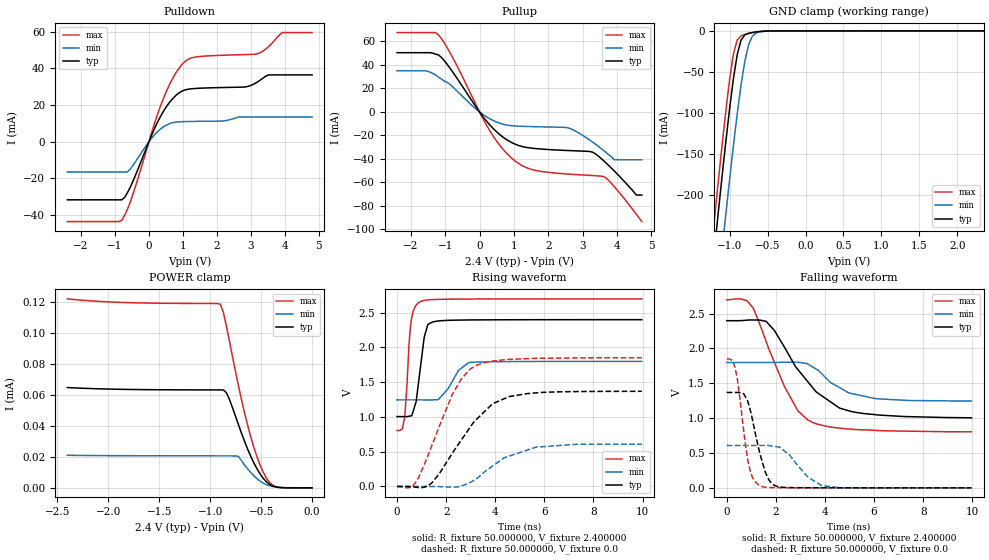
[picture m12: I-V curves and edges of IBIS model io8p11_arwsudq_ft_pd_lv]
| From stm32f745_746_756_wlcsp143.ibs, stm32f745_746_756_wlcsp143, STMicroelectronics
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|   Model io8p11_arwsudq_ft_pd_lv
[Model]  io8p11_arwsudq_ft_pd_lv
Model_type I/O
Polarity   Non-Inverting
Enable   Active-Low
Vinl =   0.720000V
Vinh =   1.680000V
Vmeas =  1.200000V
Cref =   30.000000pF
Rref =   100.000000M
Vref =   0.0V
C_comp   2.828100pF   2.774600pF   2.917100pF
[Temperature Range]   25.000000   0.125000k   -40.000000
[Pullup Reference]   2.400000V   1.800000V   2.700000V
[Pulldown Reference]   0.0V   0.0V   0.0V
[POWER Clamp Reference]   2.400000V   1.800000V   2.700000V
[GND Clamp Reference]   0.0V   0.0V   0.0V
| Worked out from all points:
|   slope of the pulldown table from 0 to 0.36 V, typ, clamps not added: 25 ohm
|   slope of the pullup table from 0 to 0.36 V, typ, clamps not added: 27.7 ohm
|   GND clamp passes 1 mA (typ) near -0.62 V on its own axis
|   rising waveform, R_fixture 50.000000, V_fixture 2.400000: 20-80 % time 296ps typ, 618ps min, 206ps max; typ from 1 V to 2.4 V
|   rising waveform, R_fixture 50.000000, V_fixture 0.0: 20-80 % time 1.73ns typ, 1.71ns min, 1.33ns max; typ from 0 V to 1.37 V
|   falling waveform, R_fixture 50.000000, V_fixture 2.400000: 20-80 % time 1.84ns typ, 1.34ns min, 1.4ns max; typ from 2.4 V to 1 V
|   falling waveform, R_fixture 50.000000, V_fixture 0.0: 20-80 % time 556ps typ, 948ps min, 410ps max; typ from 1.37 V to 0 V
[Pulldown]
|Voltage   I(typ)   I(min)   I(max)
-2.4V     -31.67mA   -16.51mA   -43.52mA
-800mV    -31.67mA   -16.51mA   -42.86mA
-480mV    -21.98mA   -13.17mA   -29.21mA
80mV      3.63mA     1.966mA    5.012mA
480mV     18.15mA    8.738mA    26.02mA
800mV     25.38mA    10.72mA    37.77mA
1.12V     28.53mA    11.02mA    44.6mA
2.8V      29.84mA    13.49mA    47.53mA
3.2V      32.65mA    13.49mA    48.03mA
3.52V     36.46mA    13.49mA    51.84mA
3.92V     36.46mA    13.49mA    59.54mA
4.8V      36.46mA    13.49mA    59.54mA
[Pullup]
|Voltage   I(typ)   I(min)   I(max)
-2.4V     50.45mA    35.08mA    67.58mA
-1.52V    50.45mA    34.74mA    67.58mA
-1.2V     48.68mA    29.86mA    65.71mA
320mV     -11.75mA   -6.207mA   -17.08mA
1.04V     -27.54mA   -11.97mA   -41.91mA
1.6V      -31.13mA   -12.58mA   -49.63mA
2.56V     -32.88mA   -13.49mA   -52.9mA
3.28V     -34.2mA    -25.53mA   -54.18mA
3.6V      -41.32mA   -32.62mA   -54.99mA
3.92V     -50.34mA   -40.8mA    -63.66mA
4.56V     -70.8mA    -40.8mA    -87.12mA
4.72V     -70.8mA    -40.8mA    -93.4mA
[GND_clamp]
|Voltage   I(typ)   I(min)   I(max)
-2.4V     -1.424A    -1.508A    -1.394A
-1.25V    -311.8mA   -402mA     -274.5mA
-1.2V     -266mA     -356.2mA   -228.4mA
-1.15V    -220.9mA   -310.9mA   -183.1mA
-1.1V     -176.9mA   -266.3mA   -139mA
-1.05V    -134.3mA   -222.6mA   -97.01mA
-950mV    -57.82mA   -139.1mA   -27.87mA
-900mV    -28.73mA   -100.5mA   -11.05mA
-850mV    -11.3mA    -65.69mA   -6.068mA
-750mV    -2.863mA   -16.61mA   -3.194mA
-600mV    -761.3uA   -1.176mA   -752.1uA
2.35V     58.09uA    37.92uA    67.25uA
[POWER_clamp]
|Voltage   I(typ)   I(min)   I(max)
-2.4V     64.71uA    21.03uA    121.9uA
-1.86V    63.55uA    20.74uA    119.6uA
-900mV    63.18uA    20.63uA    118.5uA
-870mV    63.14uA    20.63uA    113.2uA
-840mV    61.36uA    20.62uA    104.3uA
-720mV    40.37uA    20.18uA    65.28uA
-630mV    24.69uA    12.08uA    39.85uA
-540mV    12.26uA    5.907uA    20uA
-480mV    6.236uA    3.061uA    10.23uA
-420mV    2.4uA      1.365uA    3.726uA
-360mV    667.9nA    564nA      839.6nA
0V        0A         0A         0A
[Ramp]
| variable   typ   min   max
dV/dt_r  0.82110/1.72961n   0.36371/1.70409n   1.11047/1.33429n
dV/dt_f  0.83238/1.83814n   0.33264/1.35229n   1.13548/1.40034n
R_load = 50.000000
[Rising Waveform]
R_fixture= 50.000000
V_fixture= 2.400000
V_fixture_min= 1.800000
V_fixture_max= 2.700000
|time   V(typ)   V(min)   V(max)
0s        1.005V     1.245V     804.2mV
220.2ps   1.005V     1.245V     829.2mV
300.3ps   1.005V     1.246V     978.4mV
560.6ps   1.015V     1.246V     2.332V
780.8ps   1.224V     1.246V     2.607V
920.9ps   1.621V     1.246V     2.653V
1.121ns   2.165V     1.245V     2.676V
1.481ns   2.368V     1.246V     2.688V
2.923ns   2.395V     1.784V     2.696V
9.97ns    2.399V     1.799V     2.698V
[Rising Waveform]
R_fixture= 50.000000
V_fixture= 0.0
V_fixture_min= 0.0
V_fixture_max= 0.0
|time   V(typ)   V(min)   V(max)
0s        167.9uV    65.56uV    417.7uV
500.5ps   -1.047mV   52.39uV    -17.75mV
720.7ps   -7.685mV   56.75uV    40.2mV
1.401ns   46.2mV     155.1uV    573.3mV
2.262ns   483.8mV    -7.237mV   1.329V
2.623ns   669.8mV    9.988mV    1.547V
3.183ns   947mV      98.66mV    1.732V
3.904ns   1.191V     297.1mV    1.804V
5.666ns   1.346V     565.8mV    1.844V
9.97ns    1.369V     608.3mV    1.85V
[Falling Waveform]
R_fixture= 50.000000
V_fixture= 2.400000
V_fixture_min= 1.800000
V_fixture_max= 2.700000
|time   V(typ)   V(min)   V(max)
0s        2.399V     1.799V     2.698V
620.6ps   2.401V     1.799V     2.708V
1.081ns   2.409V     1.799V     2.579V
1.602ns   2.389V     1.799V     2.103V
2.342ns   2.024V     1.802V     1.461V
2.903ns   1.696V     1.802V     1.103V
3.303ns   1.523V     1.776V     974.3mV
3.804ns   1.337V     1.662V     904.6mV
5.045ns   1.098V     1.357V     842.6mV
9.97ns    1.005V     1.245V     804.2mV
[Falling Waveform]
R_fixture= 50.000000
V_fixture= 0.0
V_fixture_min= 0.0
V_fixture_max= 0.0
|time   V(typ)   V(min)   V(max)
0s        1.369V     608.3mV    1.85V
340.3ps   1.369V     608.4mV    1.727V
440.4ps   1.369V     608.3mV    1.541V
840.8ps   1.257V     608.2mV    436mV
1.041ns   989.6mV    608mV      156.6mV
1.361ns   475.6mV    608.3mV    28.91mV
1.722ns   112.6mV    607.3mV    6.038mV
2.162ns   12.06mV    581.2mV    2.818mV
3.884ns   1.268mV    32.17mV    1.078mV
9.97ns    167.9uV    65.56uV    417.7uV
